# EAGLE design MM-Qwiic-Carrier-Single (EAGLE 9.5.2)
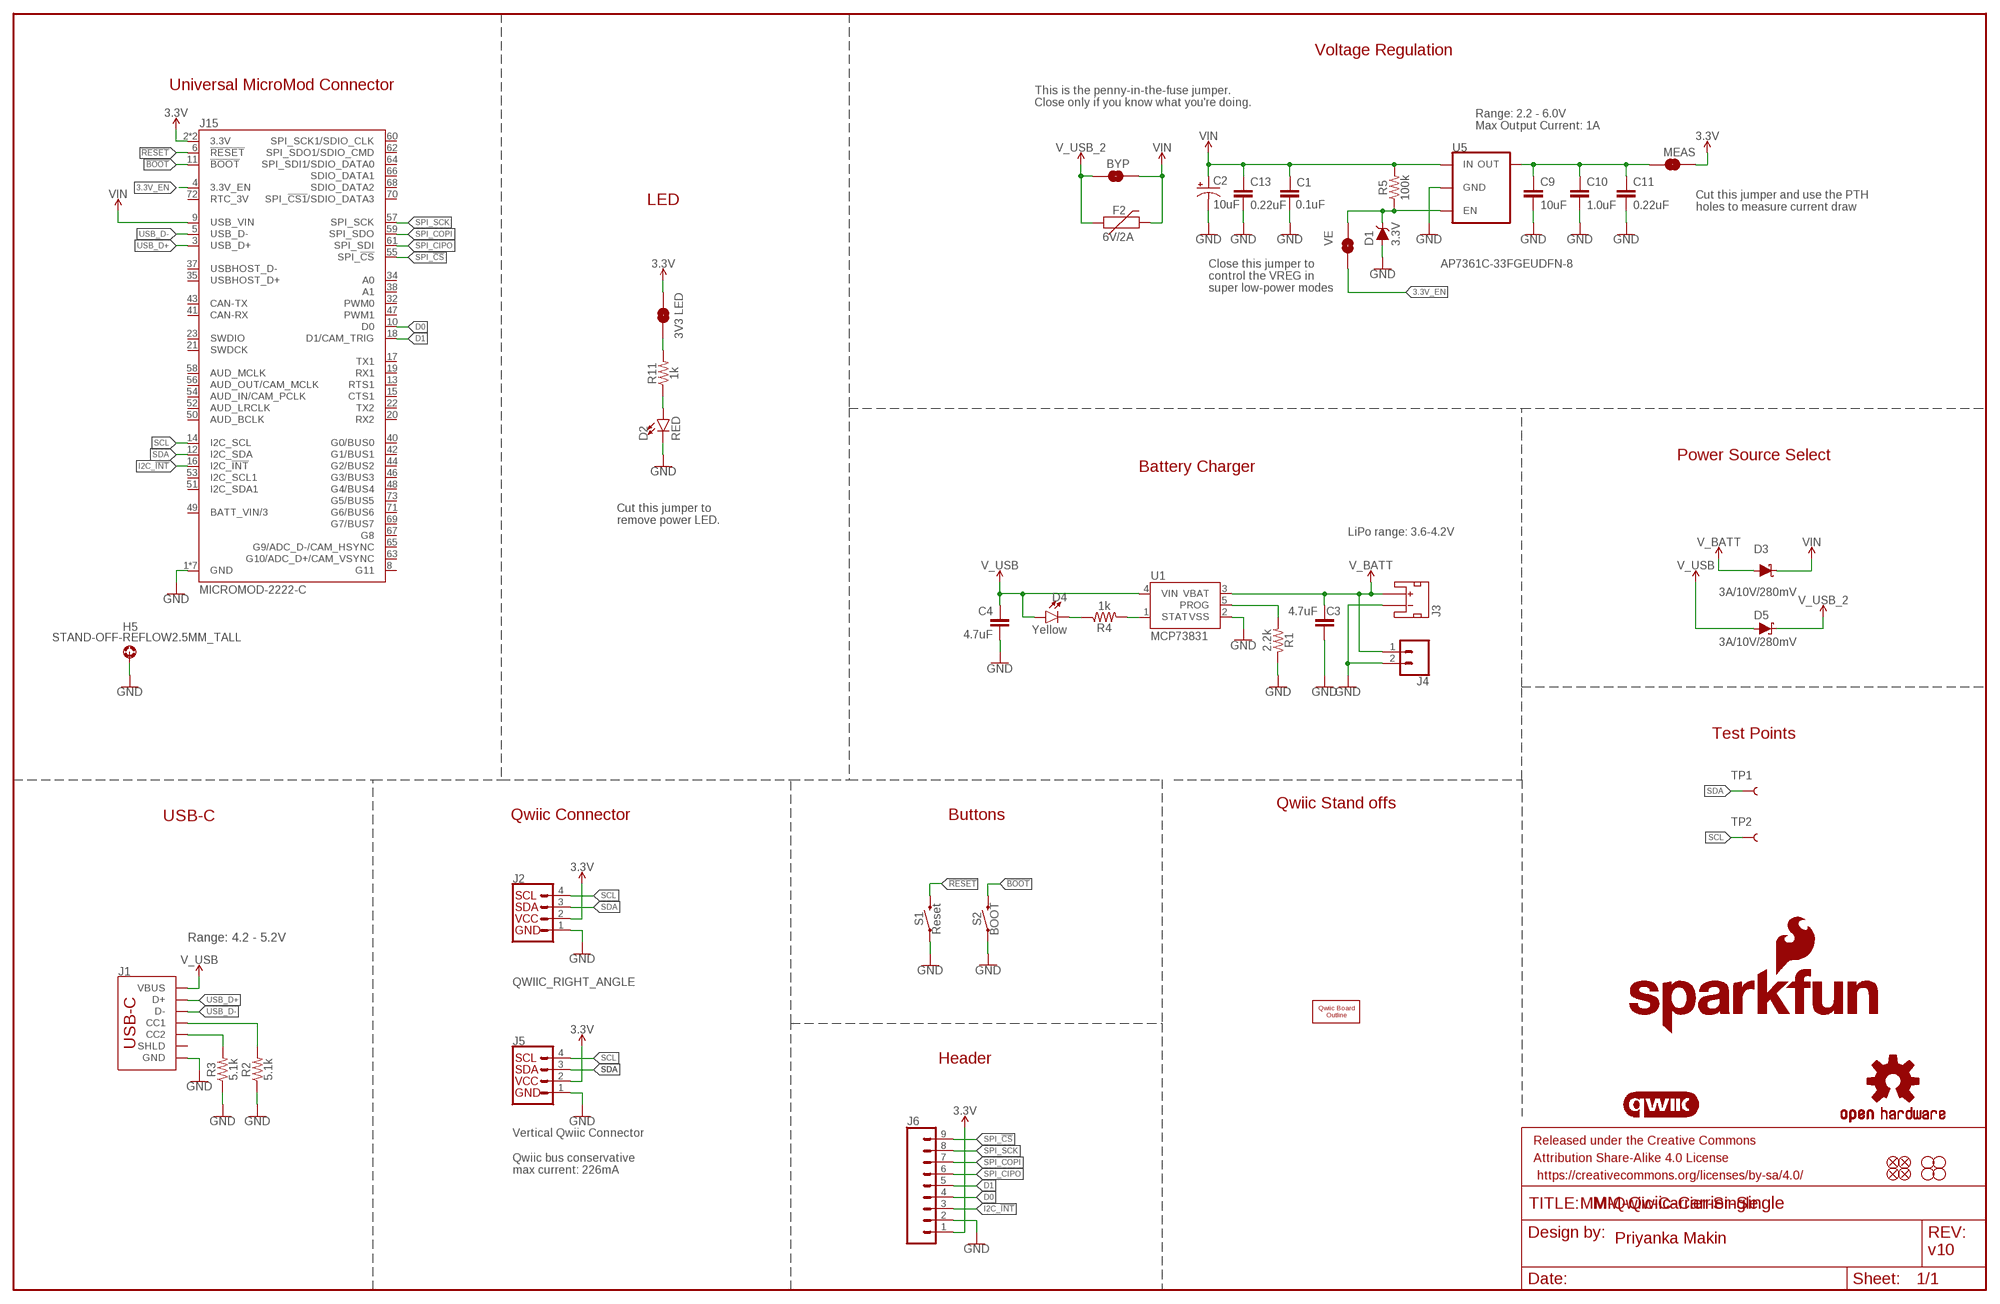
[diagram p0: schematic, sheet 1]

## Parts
BYP  JUMPER-SMT_2_NO_SILK  [SMT-JUMPER_2_NO_SILK]
C1  0.1uF  0.1UF-0603-25V-(+80/-20%)  [0603]
C2  10uF  10UF-POLAR-EIA3216-16V-10%(TANT)  [EIA3216]
C3  4.7uF  4.7UF-0603-35V-(20%)  [0603]
C4  4.7uF  4.7UF-0603-35V-(20%)  [0603]
C9  10uF  10UF-0603-6.3V-20%  [0603]
C10  1.0uF  1.0UF-0603-16V-10%  [0603]
C11  0.22uF  0.22UF-0603-25V-10%  [0603]
C13  0.22uF  0.22UF-0603-25V-10%  [0603]
D1  3.3V  DIODE-ZENER-MM3Z3V3T1G  [SOD-323]
D2  RED  LED-RED0603  [LED-0603]
D3  3A/10V/280mV  DIODE-SCHOTTKY-BAT60A  [SOD-323]
D4  Yellow  LED-YELLOW0603  [LED-0603]
D5  3A/10V/280mV  DIODE-SCHOTTKY-BAT60A  [SOD-323]
F2  6V/2A  PPTC_6V2A  [1210]
FD1  FIDUCIALUFIDUCIAL  [FIDUCIAL-MICRO]
FD2  FIDUCIALUFIDUCIAL  [FIDUCIAL-MICRO]
FD3  FIDUCIALUFIDUCIAL  [FIDUCIAL-MICRO]
FD4  FIDUCIALUFIDUCIAL  [FIDUCIAL-MICRO]
FRAME1  FRAME-LEDGER  [CREATIVE_COMMONS]
H1  STAND-OFF  [STAND-OFF]
H2  STAND-OFF  [STAND-OFF]
H3  STAND-OFF  [STAND-OFF]
H4  STAND-OFF  [STAND-OFF]
H5  STAND-OFF-REFLOW2.5MM_TALL  [STAND-OFF-REFLOW-M2.5]
J1  USB_C_2-LAYER_PADS  [USB-C-16P-2LAYER-PADS]
J2  QWIIC_RIGHT_ANGLE  QWIIC_CONNECTORJS-1MM  [JST04_1MM_RA]
J3  JST_2MM_MALE  [JST-2-SMD]
J4  CONN_021X02_NO_SILK  [1X02_NO_SILK]
J5  Vertical Qwiic Connector  QWIIC_CONNECTOR  [JST04_1MM_VERT]
J6  CONN_09NO_SILK  [1X09_NO_SILK]
J15  MICROMOD-2222-C  [M.2-CONNECTOR-E]
JP4  3V3 LED  JUMPER-SMT_2_NC_TRACE_SILK  [SMT-JUMPER_2_NC_TRACE_SILK]
JP6  VE  JUMPER-SMT_2_NO_SILK  [SMT-JUMPER_2_NO_SILK]
LOGO1  SFE_LOGO_NAME_FLAME.2_INCH  [SFE_LOGO_NAME_FLAME_.2]
LOGO2  QWIIC_LOGO_CONNECTOR  [QWIIC_5.5MM]
LOGO3  OSHW-LOGOM  [OSHW-LOGO-M]
MEAS  JUMPER-COMBO_2_NC_TRACE  [COMBO-JUMPER_2_NC_TRACE]
R1  2.2k  2.2KOHM-0603-1/10W-1%  [0603]
R2  5.1k  5.1KOHM5.1KOHM-0603-1/10W-1%  [0603]
R3  5.1k  5.1KOHM5.1KOHM-0603-1/10W-1%  [0603]
R4  1k  1KOHM-0603-1/10W-1%  [0603]
R5  100k  100KOHM-0603-1/10W-1%  [0603]
R11  1k  1KOHM-0603-1/10W-1%  [0603]
S1  Reset  MOMENTARY-SWITCH-SPST-SMD-5.2-TALL-REDUNDANT  [TACTILE_SWITCH_SMD_5.2MM]
S2  BOOT  MOMENTARY-SWITCH-SPST-SMD-5.2-TALL-REDUNDANT  [TACTILE_SWITCH_SMD_5.2MM]
TP1  TEST-POINT3X5  [PAD.03X.05]
TP2  TEST-POINT3X5  [PAD.03X.05]
U1  MCP73831  [SOT23-5]
U5  AP7361C-33FGEUDFN-8  [UDFN-8]
U$5  QWIIC_BOARD_OUTLINESTANDOFF  [QWIIC_BOARD_MOUNT_SMD_STANDOFFS]

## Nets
3.3V: J2.2 J5.2 J6.1 J15.2(3.3V) J15.74(3.3V) JP4.2 MEAS.2 MEAS.4
3.3V_EN: J15.4(3.3V_EN) JP6.1
!BOOT!: J15.11(!BOOT!) S2.3 S2.4
!RESET!: J15.6(!RESET!) S1.3 S1.4
D0: J6.4 J15.10(D0)
D1: J6.5 J15.18(D1/CAM_TRIG)
GND: C1.2 C2.- C3.2 C4.2 C9.2 C10.2 C11.2 C13.2 D1.A D2.C H5.1 J1.GND J1.GND2(GND) J2.1 J3.1(-) J4.2 J5.1 J6.2 J15.1(GND) J15.7(GND) J15.33(GND) J15.36(GND) J15.39(GND) J15.45(GND) J15.75(GND) R1.1 R2.1 R3.1 S1.1 S1.2 S2.1 S2.2 U1.2(VSS) U5.4(GND) U5.EP(GND)
I2C_!INT!: J6.3 J15.16(I2C_!INT!)
N$1: C9.1 C10.1 C11.1 MEAS.1 MEAS.3 U5.1(OUT)
N$2: R1.2 U1.5(PROG)
N$3: D4.C R4.1
N$4: JP4.1 R11.2
N$6: D2.A R11.1
N$8: R4.2 U1.1(STAT)
N$10: J1.A5(CC1) R2.2
N$11: J1.B5(CC2) R3.2
SCL: J2.4 J5.4 J15.14(I2C_SCL) TP2.P$1
SDA: J2.3 J5.3 J15.12(I2C_SDA) TP1.P$1
SPI_!CS!: J6.9 J15.55(SPI_!CS!)
SPI_CIPO: J6.6 J15.61(SPI_SDI)
SPI_COPI: J6.7 J15.59(SPI_SDO)
SPI_SCK: J6.8 J15.57(SPI_SCK)
USB_D+: J1.A6(D+) J1.B6(D+) J15.3(USB_D+)
USB_D-: J1.A7(D-) J1.B7(D-) J15.5(USB_D-)
V_BATT: C3.1 D3.A J3.2(+) J4.1 U1.3(VBAT)
V_USB: C4.1 D4.A D5.A J1.VBUS1(VBUS) J1.VBUS2(VBUS) U1.4(VIN)
V_USB_2: BYP.1 D5.C F2.1
VIN: BYP.2 C1.1 C2.+ C13.1 D3.C F2.2 J15.9(USB_VIN) R5.2 U5.8(IN)
VREG_EN: D1.C JP6.2 R5.1 U5.5(EN)
Unconnected: J1.SHLD1(SHLD) J1.SHLD2(SHLD) J1.SHLD3(SHLD) J1.SHLD4(SHLD) J3.NC1(PAD1) J3.NC2(PAD2) J15.8(G11) J15.13(RTS1) J15.15(CTS1) J15.17(TX1) J15.19(RX1) J15.20(RX2) J15.21(SWDCK) J15.22(TX2) J15.23(SWDIO) J15.32(PWM0) J15.34(A0) J15.35(USBHOST_D+) J15.37(USBHOST_D-) J15.38(A1) J15.40(G0/BUS0) J15.41(CAN-RX) J15.42(G1/BUS1) J15.43(CAN-TX) J15.44(G2/BUS2) J15.46(G3/BUS3) J15.47(PWM1) J15.48(G4/BUS4) J15.49(BATT_VIN/3) J15.50(AUD_BCLK) J15.51(I2C_SDA1) J15.52(AUD_LRCLK) J15.53(I2C_SCL1) J15.54(AUD_IN/CAM_PCLK) J15.56(AUD_OUT/CAM_MCLK) J15.58(AUD_MCLK) J15.60(SPI_SCK1/SDIO_CLK) J15.62(SPI_SDO1/SDIO_CMD) J15.63(G10/ADC_D+/CAM_VSYNC) J15.64(SPI_SDI1/SDIO_DATA0) J15.65(G9/ADC_D-/CAM_HSYNC) J15.66(SDIO_DATA1) J15.67(G8) J15.68(SDIO_DATA2) J15.69(G7/BUS7) J15.70(SPI_!CS1!/SDIO_DATA3) J15.71(G6/BUS6) J15.72(RTC_3V) J15.73(G5/BUS5)

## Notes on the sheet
- Voltage Regulation
- Universal MicroMod Connector
- This is the penny-in-the-fuse jumper.
  Close only if you know what you're doing.
- Range: 2.2 - 6.0V
  Max Output Current: 1A
- LED
- Cut this jumper and use the PTH 
  holes to measure current draw
- Close this jumper to 
  control the VREG in 
  super low-power modes
- Power Source Select
- Battery Charger
- Cut this jumper to
  remove power LED.
- LiPo range: 3.6-4.2V
- Test Points
- Qwiic Stand offs
- USB-C | Qwiic Connector | Buttons
- Range: 4.2 - 5.2V
- Header
- Qwiic bus conservative 
  max current: 226mA
- MM-Qwiic-Carrier-Single
- Priyanka Makin
- v10

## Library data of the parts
BYP JP6 = SparkFun-Jumpers:JUMPER-SMT_2_NO: Normally open jumper
C1 = SparkFun-Capacitors:0.1UF: 0.1µF ceramic capacitors; PROD_ID: CAP-00810
C2 = SparkFun-Capacitors:10UF-POLAR: 10.0µF polarized capacitors; PROD_ID: CAP-00811
C3 C4 = SparkFun-Capacitors:4.7UF: 4.7µF ceramic capacitors; PROD_ID: CAP-14106
C9 = SparkFun-Capacitors:10UF: 10.0µF ceramic capacitors; PROD_ID: CAP-11015
C10 = SparkFun-Capacitors:1.0UF: 1µF ceramic capacitors; PROD_ID: CAP-00868
C11 C13 = SparkFun-Capacitors:0.22UF: 0.22µF ceramic capacitors; PROD_ID: CAP-07822
D1 = SparkFun-DiscreteSemi:DIODE-ZENER: Zener Diode; PROD_ID: DIO-11284
D2 = SparkFun-LED:LED-RED: Red SMD LED; PROD_ID: DIO-00819
D3 D5 = SparkFun-DiscreteSemi:DIODE-SCHOTTKY: Schottky diode; PROD_ID: DIO-14072
D4 = SparkFun-LED:LED-YELLOW: Yellow SMD LED; PROD_ID: DIO-09003
F2 = SparkFun-Fuses:PPTC: Resettable Fuse PPTC; PROD_ID: RES-14313
FD1-FD4 = SparkFun-Aesthetics:FIDUCIAL: Fiducial Alignment Points
FRAME1 = SparkFun-Aesthetics:FRAME-LEDGER: Schematic Frame - Ledger
H1-H4 = SparkFun-Hardware:STAND-OFF: Stand Off
H5 = SparkFun-Hardware:STAND-OFF-REFLOW: Stand Off Reflow Compatible; PROD_ID: HW-14899
J1 = SparkFun-Connectors:USB_C: USB Type C 16Pin Connector Super Speed pins not available on the 16-pin purely SMD connector so this part is best for USB 2.0 implementations. D1 and D2 are tied together enabling D+/- no matter which way the cable is plugged into the connector. The two channel configuration pins (CC1/2) are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; PROD_ID: CONN-14122
J2 = SparkFun-Connectors:QWIIC_CONNECTOR: SparkFun I2C Standard Qwiic Connector An SMD 1mm pitch JST connector makes it easy and quick (get it? Qwiic?) to connect I2C devices to each other. The Qwiic system enables fast and solderless connection between popular platforms and various sensors and actuators. We carry 200mm, 100mm, 50mm, and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; PROD_ID: CONN-13694
J3 = SparkFun-Connectors:JST_2MM_MALE: JST 2MM MALE RA CONNECTOR Two pin, compact surface mount connector. Commonly used as a battery input connection point. We really like the solid locking feeling and high current rating on these small connectors. We use these all the time as battery connectors. Mates to single-cell LiPo batteries.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; PROD_ID: CONN-11443; SF_ID: PRT-08612
J4 = SparkFun-Connectors:CONN_02: Multi connection point. Often used as Generic Header-pin footprint for 0.1 inch spaced/style header connections
J5 = SparkFun-Connectors:QWIIC_CONNECTOR: SparkFun I2C Standard Qwiic Connector An SMD 1mm pitch JST connector makes it easy and quick (get it? Qwiic?) to connect I2C devices to each other. The Qwiic system enables fast and solderless connection between popular platforms and various sensors and actuators. We carry 200mm, 100mm, 50mm, and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; PROD_ID: CONN-14483
J6 = SparkFun-Connectors:CONN_09: Multi connection point. Often used as Generic Header-pin footprint for 0.1 inch spaced/style header connections On any of the 0.1 inch spaced packages, you can populate with these: Break Away Headers - Straight (PRT-00116) Break Away Male Headers - Right Angle (PRT-00553) Female Headers (PRT-00115)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
J15 = SparkFun-MicroMod:MICROMOD: MicroMod Connector Description: A card edge connector and mating PCB connector to allow various MicroMod Processor Boards to be coupled with various carrier boards of different capabilities. Based on the M.2 standard.; PROD_ID: CONN-14877
JP4 = SparkFun-Jumpers:JUMPER-SMT_2_NC_TRACE: Normally closed trace jumper
LOGO1 = SparkFun-Aesthetics:SFE_LOGO_NAME_FLAME: SparkFun Font Logo w/ Flame
LOGO2 = SparkFun-Aesthetics:QWIIC_LOGO: Qwiic Logos for placement on schematic and PCB. The 5.5mm silk logo is best for placing next to Qwiic connector.
LOGO3 = SparkFun-Aesthetics:OSHW-LOGO: Open-Source Hardware (OSHW) Logo
MEAS = SparkFun-Jumpers:JUMPER-COMBO_2_NC_TRACE
R1 = SparkFun-Resistors:2.2KOHM: 2.2kΩ resistor; PROD_ID: RES-08272
R2 R3 = SparkFun-Resistors:5.1KOHM; PROD_ID: RES-12083
R4 R11 = SparkFun-Resistors:1KOHM: 1kΩ resistor; PROD_ID: RES-07856
R5 = SparkFun-Resistors:100KOHM: 100kΩ resistor; PROD_ID: RES-07828
S1 S2 = SparkFun-Switches:MOMENTARY-SWITCH-SPST: Momentary Switch (Pushbutton) - SPST; PROD_ID: SWCH-14139
TP1 TP2 = SparkFun-Connectors:TEST-POINT: SparkFun Test Points
U1 = SparkFun-IC-Power:MCP73831: MCP73831T Li-Ion, Li-Pol Controller Miniature single cell, fully integrated Li-Ion, Li-polymer charge management controller Datasheet SparkFun Products: SparkFun ESP32 Thing SparkFun 9DoF Razor IMU M0; PROD_ID: IC-09995
U5 = SparkFun-IC-Power:AP7361C-33FGE: AP7361C 3.3V LDO Regulator; PROD_ID: VREG-14094
U$5 = SparkFun-Boards:QWIIC_BOARD_OUTLINE: Standard Outline of a Qwiic Board. Good for defining a spot on shields and board areas in which to mount a Qwiic Board.

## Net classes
0 default: width 0 mm, drill 0 mm
1 power: width 0.762 mm

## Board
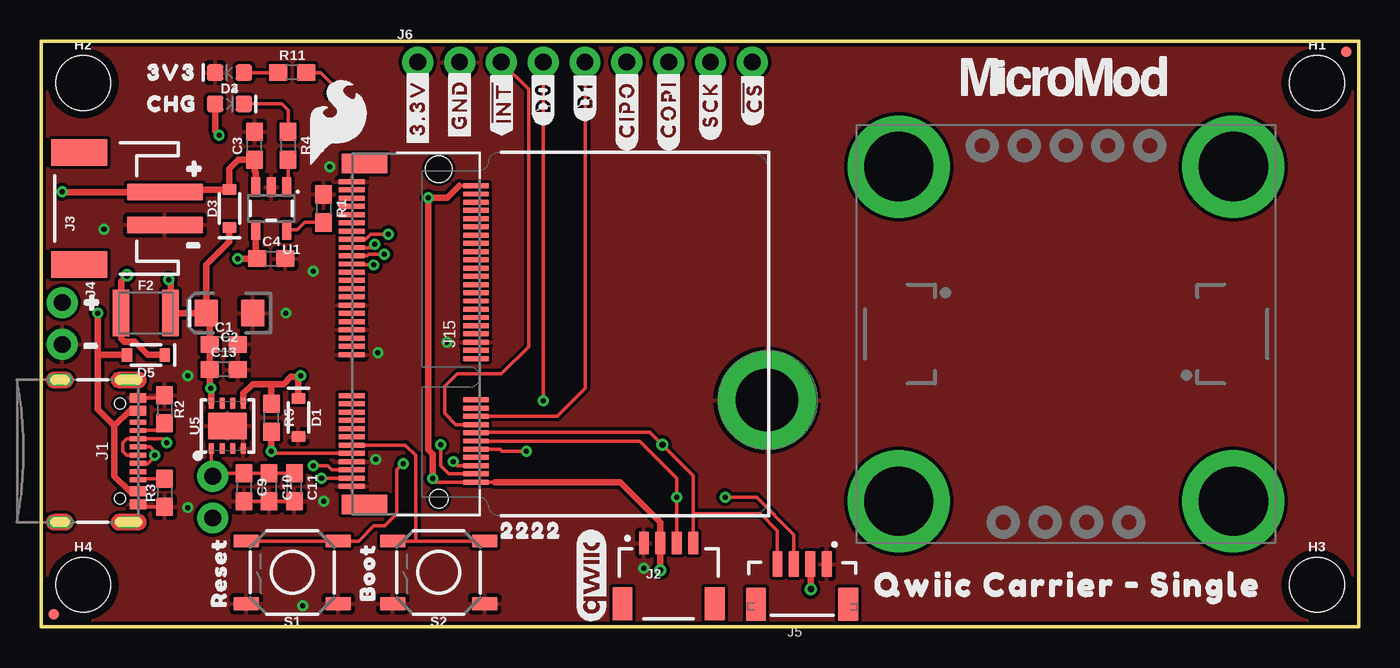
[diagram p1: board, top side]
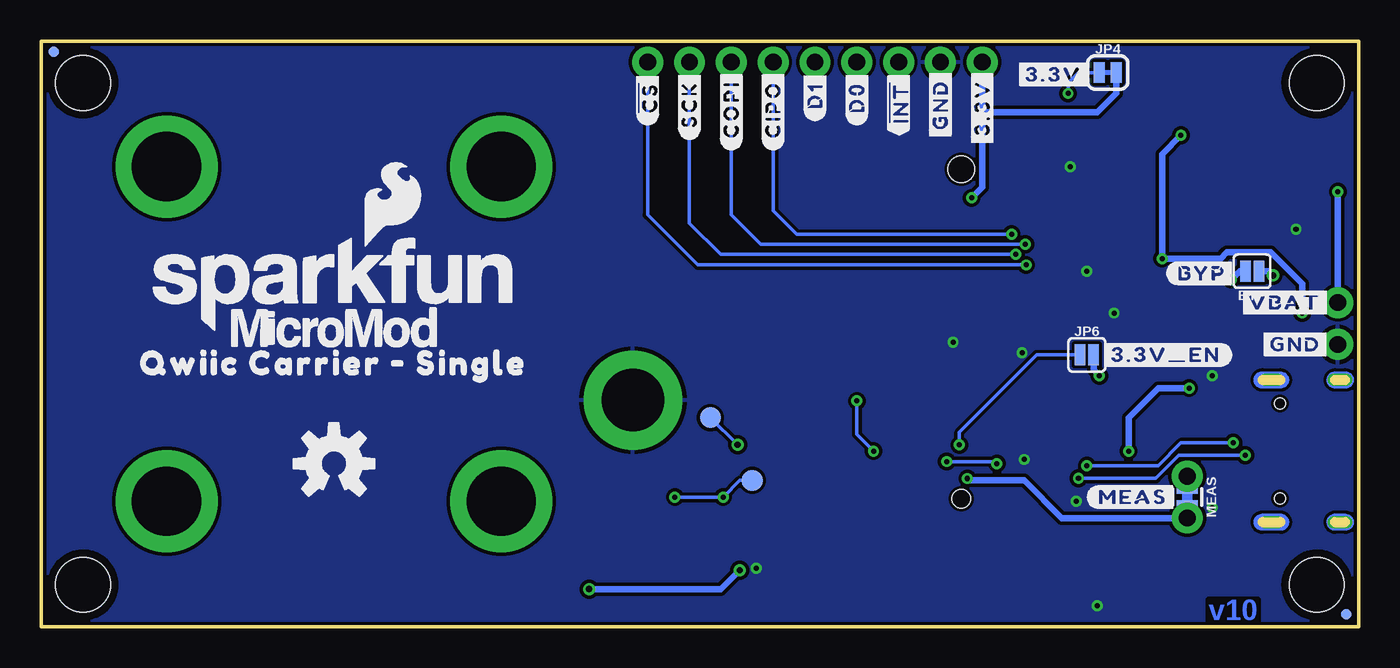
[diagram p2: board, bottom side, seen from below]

Size 80.01 x 35.56 mm. Coordinates in mm from the lower left corner, seen from the top.
Outline: 0,0 0,35.56 80.01,35.56 80.01,0 0,0
Copper layers (1*16): Top 0.035mm / dielectric 1.5mm / Bottom 0.035mm
Design rules "SparkFun-2-layer-TIGHT *": minimum track width 7mil, minimum drill 12mil, track to track 7mil, track to pad 7mil, pad to pad 7mil, via to via 7mil, smd to smd 7mil, copper to edge 7mil, drill to drill 7mil, minimum pad ring 7mil, minimum via ring 7mil, stop-mask expansion 4mil, vias tented up to drill 25mil, thermal gap 10mil

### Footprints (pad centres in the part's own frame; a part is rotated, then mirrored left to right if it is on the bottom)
SMT-JUMPER_2_NO_SILK = smd 0.635 x 1.27: 1 -0.406,0; 2 0.406,0
0603 = smd 1.1 x 1: 1 -0.85,0; 2 0.85,0
EIA3216 = smd 1.4 x 1.6: + 1.4,0; - -1.4,0
SOD-323 = smd 0.63 x 0.83: A 1.15,0; C -1.15,0
LED-0603 = smd 1 x 1: A -0.877,0; C 0.877,0
1210 = smd 1 x 2.8: 1 -1.5,0; 2 1.5,0
FIDUCIAL-MICRO = smd 0.635 x 0.635: 1 0,0
STAND-OFF = hole 3.302: 0,0
STAND-OFF-REFLOW-M2.5 = drill 3.8 pad 6: 1 0,0
USB-C-16P-2LAYER-PADS = smd 0.3 x 1: A5 -1.25,-0.34; A6 -0.25,-0.34; A7 0.25,-0.34; A8 1.25,-0.34; B5 1.75,-0.34; B6 0.75,-0.34; B7 -0.75,-0.34; B8 -1.75,-0.34 | smd 0.6 x 1: GND -3.225,-0.34; GND2 3.225,-0.34; VBUS1 -2.45,-0.34; VBUS2 2.45,-0.34 | drill 0.4 pad 0.6 long: SHLD1 -4.318,-0.915; SHLD2 4.318,-0.915; SHLD3 -4.318,-5.095; SHLD4 4.318,-5.095 | hole 0.65: -2.89,-1.445; 2.89,-1.445
JST04_1MM_RA = smd 0.6 x 1.35: 1 -1.5,0; 2 -0.5,0; 3 0.5,0; 4 1.5,0 | smd 1.2 x 2: NC1 2.8,-3.675; NC2 -2.8,-3.675
JST-2-SMD = smd 1 x 4.6: 1 -1,-3.7; 2 1,-3.7 | smd 1.6 x 3.4: NC1 -3.4,1.5; NC2 3.4,1.5
1X02_NO_SILK = drill 1.016 pad 1.88: 1 0,0; 2 2.54,0
JST04_1MM_VERT = smd 0.6 x 1.55: 1 -1.478,0.775; 2 -0.478,0.775; 3 0.522,0.775; 4 1.522,0.775 | smd 1.2 x 2: NC1 -2.778,3.2; NC2 2.822,3.2
1X09_NO_SILK = drill 1.016 pad 1.88: 1 0,0; 2 2.54,0; 3 5.08,0; 4 7.62,0; 5 10.16,0; 6 12.7,0; 7 15.24,0; 8 17.78,0; 9 20.32,0
M.2-CONNECTOR-E = smd 0.3 x 1.55: 1 9.25,-5.275; 2 9,2.275; 3 8.75,-5.275; 4 8.5,2.275; 5 8.25,-5.275; 6 8,2.275; 7 7.75,-5.275; 8 7.5,2.275; 9 7.25,-5.275; 10 7,2.275; 11 6.75,-5.275; 12 6.5,2.275; 13 6.25,-5.275; 14 6,2.275; 15 5.75,-5.275; 16 5.5,2.275; 17 5.25,-5.275; 18 5,2.275; 19 4.75,-5.275; 20 4.5,2.275; 21 4.25,-5.275; 22 4,2.275; 23 3.75,-5.275; 32 1.5,2.275; 33 1.25,-5.275; 34 1,2.275; 35 0.75,-5.275; 36 0.5,2.275; 37 0.25,-5.275; 38 0,2.275; 39 -0.25,-5.275; 40 -0.5,2.275; 41 -0.75,-5.275; 42 -1,2.275; 43 -1.25,-5.275; 44 -1.5,2.275; 45 -1.75,-5.275; 46 -2,2.275; 47 -2.25,-5.275; 48 -2.5,2.275; 49 -2.75,-5.275; 50 -3,2.275; 51 -3.25,-5.275; 52 -3.5,2.275; 53 -3.75,-5.275; 54 -4,2.275; 55 -4.25,-5.275; 56 -4.5,2.275; 57 -4.75,-5.275; 58 -5,2.275; 59 -5.25,-5.275; 60 -5.5,2.275; 61 -5.75,-5.275; 62 -6,2.275; 63 -6.25,-5.275; 64 -6.5,2.275; 65 -6.75,-5.275; 66 -7,2.275; 67 -7.25,-5.275; 68 -7.5,2.275; 69 -7.75,-5.275; 70 -8,2.275; 71 -8.25,-5.275; 72 -8.5,2.275; 73 -8.75,-5.275; 74 -9,2.275; 75 -9.25,-5.275 | smd 1.2 x 2.75: A1 10.35,-4.5; A2 -10.35,-4.5 | hole 1.1: 10,0 | hole 1.6: -10,0
SMT-JUMPER_2_NC_TRACE_SILK = smd 0.66 x 1.27: 1 -0.521,0; 2 0.521,0
COMBO-JUMPER_2_NC_TRACE = smd 0.635 x 1.27: 1 -0.508,0; 2 0.508,0 | drill 1.016 pad 1.88: 3 -1.27,0; 4 1.27,0
TACTILE_SWITCH_SMD_5.2MM = smd 1.524 x 0.762: 1 -2.794,1.905; 2 2.794,1.905; 3 -2.794,-1.905; 4 2.794,-1.905
PAD.03X.05 = smd 1.27 x 1.27: P$1 0,0
SOT23-5 = smd 0.55 x 1.2: 1 -0.95,-1.3; 2 0,-1.3; 3 0.95,-1.3; 4 0.95,1.3; 5 -0.95,1.3
UDFN-8 = smd 0.3 x 0.65: 1 -0.975,-1.375; 2 -0.325,-1.375; 3 0.325,-1.375; 4 0.975,-1.375; 5 0.975,1.375; 6 0.325,1.375; 7 -0.325,1.375; 8 -0.975,1.375 | smd 2.35 x 1.6: EP 0,0
QWIIC_BOARD_MOUNT_SMD_STANDOFFS = drill 4.216 pad 6.198: 1 -10.16,10.16; 2 10.16,10.16; 3 -10.16,-10.16; 4 10.16,-10.16

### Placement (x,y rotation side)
BYP  6.48,21.59 180 bottom
C1  11.09,17.14 0 top
C2  11.43,19.05 180 top
C3  12.95,29.21 90 top
C4  13.97,22.35 0 top
C9  12.32,8.47 270 top
C10  13.84,8.47 270 top
C11  15.37,8.47 270 top
C13  11.09,15.62 0 top
D1  15.62,12.7 270 top
D2  11.43,33.66 180 top
D3  11.43,25.4 90 top
D4  11.43,31.75 0 top
D5  6.35,16.51 180 top
F2  6.35,19.05 0 top
FD1  0.76,0.76 0 top
FD2  79.25,34.92 0 top
FD3  0.76,0.76 0 bottom
FD4  79.25,34.92 0 bottom
FRAME1  not placed on the board
H1  77.47,33.02 0 top
H2  2.54,33.02 0 top
H3  77.47,2.54 0 top
H4  2.54,2.54 0 top
H5  44.07,13.76 0 top
J1  6.22,10.67 270 top
J2  38.1,5.08 0 top
J3  3.81,25.4 90 top
J4  1.27,19.68 270 top
J5  46.23,4.57 180 top
J6  22.86,34.29 0 top
J15  24.13,17.78 270 top
JP4  15.24,33.66 0 bottom
JP6  16.51,16.51 0 bottom
LOGO1  62.23,20.83 0 bottom
LOGO2  33.4,3.11 90 top
LOGO3  62.23,9.91 0 bottom
MEAS  10.41,7.87 270 bottom
R1  17.14,25.4 270 top
R2  7.49,13.21 270 top
R3  7.49,8.13 90 top
R4  14.99,29.21 270 top
R5  13.97,12.7 270 top
R11  15.24,33.66 0 top
S1  15.24,3.3 180 top
S2  24.13,3.3 180 top
TP1  36.83,8.89 0 bottom
TP2  39.37,12.7 0 bottom
U1  13.97,25.4 180 top
U5  11.3,12.19 0 top
U$1  [#3#3V_EN#0]  15.75,16.51 0 bottom
U$2  [QWIIC_CARRIER_#_SINGLE0]  49.53,2.54 0 top
U$3  [3V30]  5.71,33.66 0 top
U$4  [CHG0]  5.71,31.75 0 top
U$5  62.23,17.78 0 top
U$6  [#3#3V#0]  20.95,33.53 0 bottom
U$7  [#BYP#0]  11.68,21.46 0 bottom
U$8  [#GND#0]  25.4,29.46 90 top
U$9  [#MEAS#0]  16.51,7.87 0 bottom
U$11  [#0]  1.52,19.68 0 top
U$12  [#VBAT#0]  7.37,19.68 0 bottom
U$14  [#GND#0]  25.4,29.46 90 bottom
U$15  [##INT##0]  27.94,29.84 90 top
U$16  [##INT##0]  27.94,29.84 90 bottom
U$17  [#D0#0]  30.48,30.48 90 top
U$18  [#D0#0]  30.48,30.48 90 bottom
U$19  [QWIIC_CARRIER_#_SINGLE0]  75.06,16 0 bottom
U$20  [#D1#0]  33.02,30.73 90 top
U$21  [#D1#0]  33.02,30.73 90 bottom
U$22  [#CIPO#0]  35.56,28.96 90 top
U$23  [#CIPO#0]  35.56,28.96 90 bottom
U$24  [#COPI#0]  38.1,28.96 90 top
U$25  [#COPI#0]  38.1,28.96 90 bottom
U$26  [#SCK#0]  40.64,29.59 90 top
U$27  [#SCK#0]  40.64,29.59 90 bottom
U$28  [##CS##0]  43.18,30.48 90 top
U$29  [##CS##0]  43.18,30.48 90 bottom
U$30  [RESET0]  10.79,0.51 90 top
U$31  [BOOT0]  19.81,0.89 90 top
U$32  [#0]  7.75,27.81 0 top
U$33  [#GND#0]  6.1,17.14 0 bottom
U$34  [22220]  27.18,5.84 0 top
U$35  [#3#3V#0]  22.86,29.08 90 top
U$36  [#0]  1.14,17.4 0 top
U$37  [#0]  7.37,23.5 0 top
U$38  [#3#3V#0]  22.86,29.08 90 bottom
U$44  [SFE_LOGO_FLAME_.2]  18.03,30.61 0 top
U$67  [MICROMOD_LOGO_.5]  62.1,33.4 0 top
U$68  [MICROMOD_LOGO_.5]  62.23,18.16 0 bottom

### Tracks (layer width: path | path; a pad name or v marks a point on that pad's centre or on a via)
3.3V  (via drill 0.3, 0.38)
  Top 0.203: v23.76,9 23.99,8.78 J15.2 27.54,8.78 | J15.74 25.38,26.78
  Top 0.406: v23.76,9 23.76,10.48 23.51,10.74 v23.51,26.05 24.65,26.05 25.38,26.78 | v37.59,3.43 v37.6,3.44 J2.2 37.6,6.34 35.16,8.78 27.54,8.78 | v46.74,2.29 46.74,3.77 J5.2
  Bottom 0.203: MEAS.2 MEAS.4 | v23.76,9 23.65,8.89
  Bottom 0.406: MEAS.4 18.03,6.6 20.32,8.89 23.65,8.89 | JP4.2 14.72,32.4 15.88,31.24 22.86,31.24 | v37.59,3.43 38.73,2.29 v46.74,2.29 | J6.1 22.86,31.24 | 22.86,31.24 22.86,26.7 v23.51,26.05
3.3V_EN  (via drill 0.3)
  Top 0.203: J15.4 24.76,9.28 24.26,9.78 v24.26,11.05
  Bottom 0.203: v24.26,11.05 24.26,11.81 19.56,16.51 JP6.1
!BOOT!
  Top 0.203: S2.4 22.73,5.21 | 22.73,5.21 S2.3 | 22.73,5.21 22.73,10.41 22.12,11.03 J15.11
!RESET!  (via drill 0.3)
  Top 0.203: v25.02,10.03 v25.02,10.02 25.26,9.78 J15.6 | v21.97,9.91 21.59,9.53 21.59,6.86 20.85,6.12 20.2,6.12 19.29,5.21 S1.3 S1.4
  Bottom 0.203: v21.97,9.91 22.1,10.03 v25.02,10.03
D0  (via drill 0.3)
  Top 0.203: v29.46,10.67 27.97,10.67 27.86,10.78 J15.10 | J6.4 v30.48,13.72
  Bottom 0.203: v30.48,13.72 30.48,11.68 v29.46,10.67
D1
  Top 0.203: J15.18 31.32,12.78 32.77,14.22 33.02,14.48 J6.5
GND  (via drill 0.3)
  Top 0.203: J1.GND 7.33,13.89 R2.1 | J1.GND2 6.05,7.28 R3.1 | C9.2 C10.2 C11.2
  other vias: 17.53,27.94 3.81,24.13 16.51,21.59 14.86,19.05 8.89,15.24 8.89,7.24 15.88,1.27 17.14,7.62 20.32,10.16 36.58,3.56 20.45,16.64 24.64,17.27
  pour Top (isolate 0.203): 0,35.56 0,0 80.01,0 80.01,35.56
  pour Bottom (isolate 0.203): 0,35.56 0,0 80.01,0 80.01,35.56
I2C_!INT!
  Top 0.203: J15.16 25.18,12.28 24.51,12.95 24.51,14.61 25.27,15.37 27.94,15.37 29.59,17.02 29.59,31.75 29.59,32.64 J6.3
N$1
  Top 0.203: C11.1 C10.1 C9.1 11.3,9.32 11.13,9.14 MEAS.3 10.33,9.23 U5.1
  Bottom 0.203: MEAS.1 MEAS.3
N$2
  Top 0.203: U1.5 15.55,24.1 16,24.55 R1.2
N$3
  Top 0.203: D4.C 14.61,31.75 14.99,31.37 R4.1
N$4  (via drill 0.3)
  Top 0.203: v17.65,32.38 17.65,32.98 16.98,33.66 R11.2
  Bottom 0.203: v17.65,32.38 17.65,33.03 17.03,33.66 JP4.1
N$6
  Top 0.203: D2.A R11.1
N$8
  Top 0.203: U1.1 14.99,26.77 R4.2
N$10
  Top 0.203: J1.A5 7.05,11.92 R2.2
N$11
  Top 0.203: J1.B5 5.94,8.98 R3.2
SCL  (via drill 0.38)
  Top 0.203: J2.4 39.6,6.86 | 39.6,6.86 39.6,9.17 v37.72,11.05 36.96,11.81 26.44,11.81 J15.14 | J5.4 44.71,5.84 43.69,6.86 39.6,6.86
  Bottom 0.203: TP2.P$1 v37.72,11.05
SDA  (via drill 0.3)
  Top 0.203: J2.3 v38.6,7.87 38.6,9.03 36.34,11.28 J15.12 | J5.3 45.71,5.6 43.43,7.87 v41.53,7.87
  Bottom 0.203: v41.53,7.87 v38.6,7.87 37.58,8.89 TP1.P$1
SPI_!CS!  (via drill 0.3)
  Top 0.203: v20.19,21.97 18.91,21.97 J15.55
  Bottom 0.203: v20.19,21.97 40.13,21.97 43.18,25.02 J6.9
SPI_CIPO  (via drill 0.3)
  Top 0.203: J15.61 19.69,23.53 20,23.84 v21.08,23.84
  Bottom 0.203: v21.08,23.84 34.12,23.84 35.56,25.27 J6.6
SPI_COPI  (via drill 0.3)
  Top 0.203: v20.25,23.23 20.05,23.03 J15.59
  Bottom 0.203: v20.25,23.23 36.31,23.23 38.1,25.02 J6.7
SPI_SCK  (via drill 0.3)
  Top 0.203: v20.83,22.62 19.89,22.62 19.8,22.53 J15.57
  Bottom 0.203: v20.83,22.62 20.83,22.61 38.73,22.61 40.64,24.51 J6.8
USB_D+  (via drill 0.3)
  Top 0.203: J1.A6 6.61,10.92 6.86,10.67 6.86,10.45 v6.89,10.41 6.89,10.32 6.48,9.91 5.89,9.91 J1.B6 | J15.3 v17.03,9.03 v17.02,9.02
  Bottom 0.203: v17.02,9.02 12.32,9.02 10.92,10.41 v6.89,10.41
USB_D-  (via drill 0.3)
  Top 0.203: J1.A7 5.2,10.42 4.95,10.67 4.95,11.18 5.2,11.42 J1.B7 7.38,11.42 v7.62,11.17 | J15.5 17.65,9.53 17.4,9.78 v16.51,9.78
  Bottom 0.203: v7.62,11.17 10.79,11.17 12.19,9.78 v16.51,9.78
V_BATT  (via drill 0.3)
  Top 0.406: U1.3 13.02,27.59 12.95,27.66 C3.1 11.98,28.36 11.43,27.81 D3.A 7.66,26.55 J3.2 1.29,26.4 v1.27,26.42
  Bottom 0.406: v1.27,26.42 J4.1
V_USB  (via drill 0.3)
  Top 0.406: J1.VBUS2 5.37,8.22 4.45,9.14 4.45,12.19 | J1.VBUS1 5.37,13.12 4.45,12.19 | 4.45,12.19 3.43,13.21 3.43,16.51 | v3.43,19.05 3.43,16.51 | v11.94,22.35 C4.1 13.02,22.45 U1.4 | D4.A 10.55,30.09 v10.79,29.84 | D5.A 3.43,16.51
  Bottom 0.406: v3.43,19.05 3.43,20.83 5.33,22.73 8,22.73 8.38,22.35 v11.94,22.35 11.94,28.7 v10.79,29.84
V_USB_2  (via drill 0.38)
  Top 0.406: D5.C 6.47,16.51 5.67,17.31 5.05,17.31 4.85,17.5 F2.1 4.85,20.98 v5.21,21.34
  Bottom 0.406: v5.21,21.34 5.46,21.59 BYP.1
VIN  (via drill 0.3)
  Top 0.203: v13.97,10.67 13.97,10.66 14.1,10.53 J15.9
  Top 0.406: C2.+ F2.2 7.85,20.98 v7.75,21.08 | C2.+ 10.24,18.84 C1.1 C13.1 10.24,14.55 v10.3,14.49 10.33,14.46 U5.8 | R5.2 v13.97,10.67 | D3.C 11.43,23.37 10.03,21.97 C2.+
  Bottom 0.406: v7.75,21.08 7.24,21.59 BYP.2 | v10.3,14.49 12.18,14.49 13.97,12.7 v13.97,10.67
VREG_EN  (via drill 0.3)
  Top 0.406: D1.C 15.62,15.11 15.68,15.18 | 15.68,15.18 v15.75,15.24 | R5.1 13.97,14.73 13.96,14.74 | U5.5 12.28,14.18 12.84,14.74 13.96,14.74 | 13.96,14.74 14.72,14.74 15.16,15.18 15.68,15.18
  Bottom 0.406: v15.75,15.24 16.1,15.6 JP6.2

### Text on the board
Bottom: v10
Measures: in | in | in | in | in | in
tDocu: Priyanka Makin

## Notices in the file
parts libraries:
SparkFun-Aesthetics: Licensing: Creative Commons ShareAlike 4.0 International - https://creativecommons.org/licenses/by-sa/4.0
SparkFun-Aesthetics: Released under the Creative Commons Attribution Share-Alike 4.0 License
SparkFun-Aesthetics: https://creativecommons.org/licenses/by-sa/4.0
